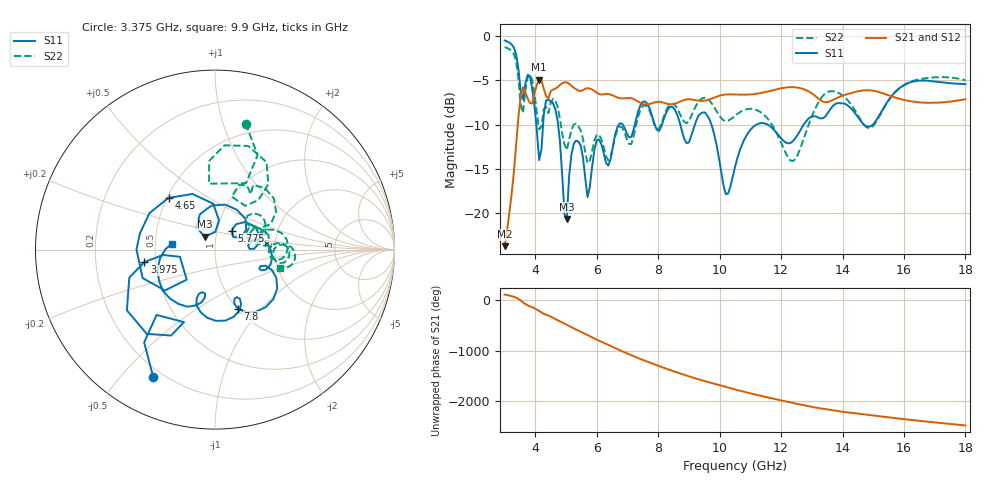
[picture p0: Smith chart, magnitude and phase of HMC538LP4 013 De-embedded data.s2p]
! Chelmsford, MA 01824
! http://www.hittite.com
! Tel: 978-250-3343
! Fax: 978-250-3373
! Device  :  HMC538LP4
! Description:  600 Analog Phase Shifter
! Frequency  :  6.0 GHz - 15.0 GHz
! Package  :  LP4  - 4x4 mm Quad Flatpack No-Lead (QFN) Plastic Package: 24 pin
! Ports  :  2 RF, 1 DC
!  Pin  3  = Rfin  = Port 1
!  Pin  16  = Rfout = Port 2
!  pin  21  = vCTL
! Voltages:  VCTL  = 0 to 5.0 Volts
! Currents :  Vb(V)  Vd(V)  Ib(mA)  Id(mA)
!  0.00  1.30  0.000000	0.487576
! Data:  The device was measured on evaluation board 111296-1.
!  Data was collected using a calibrated network analyzer.
!  The evaluation circuit board was modeled and simulated.This was use
!  to removed the evaluation board circuit from the measured data.
!  The reference plane is the center of the package pin.
! Misc:  Lot #
!Date Measured:  03 - 11 -2009
! Date:  03 - 17 -2009
! Note:
!  Hittite Microwave supplies this data as a sample of measured data at the
!  package pin for this package product.  Your particular data for this product
!  may vary.
!  Data was taken at 25 degrees C.
!  Hittite Microwave reserves the right to change this data at anytime.
# MHz S MA R 50
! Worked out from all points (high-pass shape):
!   201 points, 3 GHz to 18 GHz, reference 50 ohm
!   highest |S21| = -4.90 dB at 4.125 GHz (marker M1); lowest = -23.7 dB at 3 GHz (marker M2)
!   |S21| within 3 dB of the highest: 3.488 GHz to end of sweep
!   lowest |S11| = -20.7 dB at 5.025 GHz (marker M3), VSWR 1.20, Z = 44.1 + j6.4 ohm
!   |S11| at or under -10 dB: 4.741 GHz to 6.722 GHz (1.982 GHz wide, 34.6 % of centre); 9.733 GHz to 11.2 GHz (1.466 GHz wide, 14 % of centre); 11.56 GHz to 12.74 GHz (1.172 GHz wide, 9.65 % of centre)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
!   |S22| runs from -14.4 to -1.2 dB; largest |S21 - S12| = 0.0014
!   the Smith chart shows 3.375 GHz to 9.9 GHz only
!   S11 on the Smith chart (normalised r, x): 3.375 GHz: 0.16, -0.62; 3.975 GHz: 0.43, -0.07; 4.65 GHz: 0.51, +0.35; 5.775 GHz: 1.18, +0.25; 7.8 GHz: 1.01, -0.76; 9.9 GHz: 0.61, +0.04
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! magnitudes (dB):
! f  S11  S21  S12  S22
! 3 GHz  -0.5  -23.7  -23.7  -1.2
! 3.375 GHz  -2.1  -12.3  -12.3  -2.8
! 3.6 GHz  -7.1  -5.8  -5.8  -8.7
! 3.975 GHz  -8.0  -6.4  -6.4  -6.5
! 4.125 GHz  -14.0  -4.9  -4.9  -10.5
! 4.35 GHz  -7.3  -6.8  -6.8  -8.0
! 4.65 GHz  -8.2  -5.9  -5.9  -7.2
! 5.025 GHz  -20.7  -5.2  -5.2  -12.9
! 5.25 GHz  -12.2  -5.8  -5.8  -10.0
! 5.55 GHz  -13.7  -6.1  -6.1  -11.6
! 5.775 GHz  -17.0  -5.9  -5.9  -14.1
! 6 GHz  -11.8  -6.4  -6.4  -11.1
! 7.8 GHz  -9.0  -7.6  -7.6  -9.2
! 8.025 GHz  -10.7  -7.4  -7.4  -10.5
! 9.9 GHz  -12.3  -6.8  -6.9  -8.5
! 10.2 GHz  -17.8  -6.6  -6.6  -9.6
! 10.5 GHz  -14.8  -6.6  -6.6  -9.0
! 11.25 GHz  -9.9  -6.5  -6.5  -8.4
! 12.38 GHz  -11.9  -5.8  -5.8  -14.1
! 13.05 GHz  -9.0  -6.6  -6.6  -8.7
! 15.53 GHz  -7.1  -6.7  -6.7  -7.1
! 18 GHz  -5.4  -7.1  -7.1  -5.0
